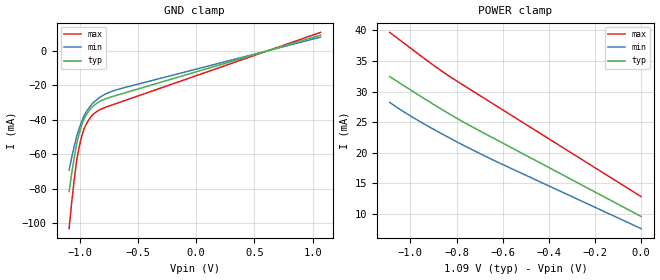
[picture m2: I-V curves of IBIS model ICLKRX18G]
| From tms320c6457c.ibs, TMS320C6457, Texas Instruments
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|   Model Cell ICLKRX18G
|  Cell operated at 1.09(nom)
|  BUFFER WITH +/- 5% VDDS
[Model]   ICLKRX18G
Model_type   Input
Polarity   Non-Inverting
Vinl =  0.545
Vinh =  0.98
C_comp   0.222256p   0.1052251p   0.4637717p
[Model Spec]
Vinl   0.545   0.5225   0.5775
Vinh   0.98   0.98   0.98
[Temperature Range]   25   125   -40
[Voltage Range]   1.09   1.045   1.155
[POWER_clamp]
|   voltage   I(typ)   I(min)   I(max)
-1.09V    32.43mA    28.21mA    39.65mA
-990.9mV  30.04mA    25.81mA    36.82mA
-891.8mV  27.71mA    23.67mA    34.06mA
-825.8mV  26.21mA    22.32mA    32.35mA
-726.7mV  24.12mA    20.38mA    29.98mA
-9.548fV  9.603mA    7.618mA    12.84mA
[GND_clamp]
|   voltage   I(typ)   I(min)   I(max)
-1.09V    -81.73mA   -69.2mA    -103.3mA
-1.068V   -71.32mA   -62.03mA   -88.25mA
-1.046V   -61.94mA   -55.43mA   -74.83mA
-1.024V   -53.6mA    -49.41mA   -63.06mA
-1.002V   -47.67mA   -44.7mA    -55.32mA
-979.9mV  -42.79mA   -40.61mA   -49.18mA
-957.9mV  -38.96mA   -37.15mA   -44.62mA
-913.8mV  -34.36mA   -32.54mA   -39.34mA
-869.8mV  -31.32mA   -29.33mA   -36.11mA
-781.7mV  -27.98mA   -25.18mA   -32.9mA
-671.6mV  -25.57mA   -22.38mA   -30.25mA
1.068V    9.163mA    8.018mA    10.79mA
